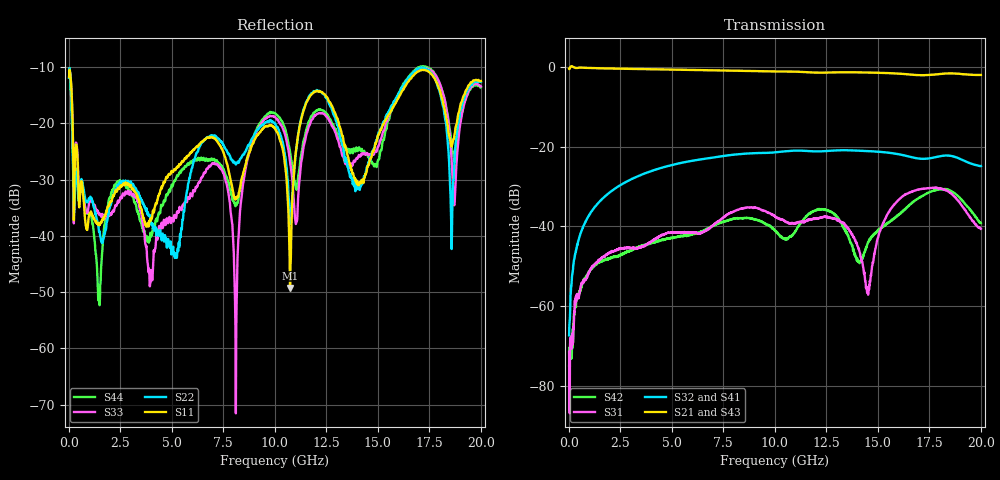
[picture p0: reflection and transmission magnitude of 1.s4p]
!Keysight Technologies,N5225A,MY51451420,A.10.40.12
!Date: Tuesday, October 13, 2015 09:32:39
!Correction: S11(Full 4 Port(1,2,3,4))
!S12(Full 4 Port(1,2,3,4))
!S13(Full 4 Port(1,2,3,4))
!S14(Full 4 Port(1,2,3,4))
!S21(Full 4 Port(1,2,3,4))
!S22(Full 4 Port(1,2,3,4))
!S23(Full 4 Port(1,2,3,4))
!S24(Full 4 Port(1,2,3,4))
!S31(Full 4 Port(1,2,3,4))
!S32(Full 4 Port(1,2,3,4))
!S33(Full 4 Port(1,2,3,4))
!S34(Full 4 Port(1,2,3,4))
!S41(Full 4 Port(1,2,3,4))
!S42(Full 4 Port(1,2,3,4))
!S43(Full 4 Port(1,2,3,4))
!S44(Full 4 Port(1,2,3,4))
!S4P File: Measurements: <S11,S12,S13,S14>,
!<S21,S22,S23,S24>,
!<S31,S32,S33,S34>,
!<S41,S42,S43,S44>:
# Hz S  dB  R 50
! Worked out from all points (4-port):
!   1999 points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, 20 MHz to 20 GHz, reference 50 ohm
!   strongest paths, dB at 20 MHz, 5.01 GHz, 10.01 GHz, 15.01 GHz, 20 GHz:
!     S21: -0.5, -0.7, -1.2, -1.5, -2.0
!     S43: -0.5, -0.7, -1.2, -1.5, -1.9
!     S32: -67.4, -24.6, -21.5, -21.3, -24.9
!     S41: -68.7, -24.6, -21.5, -21.3, -24.9
!     S31: -71.5, -41.6, -37.6, -42.8, -40.6
!     S42: -74.9, -43.0, -41.0, -41.1, -39.2
!   lowest |S11| = -49.3 dB at 10.74 GHz (marker M1), VSWR 1.01, Z = 50.1 - j0.322 ohm
!   |S11| at or under -10 dB: start of sweep to end of sweep
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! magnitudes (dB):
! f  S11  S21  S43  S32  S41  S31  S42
! 20 MHz  -11.8  -0.5  -0.5  -67.4  -68.7  -71.5  -74.9
! 1.47 GHz  -38.1  -0.4  -0.4  -34.0  -34.0  -48.6  -49.1
! 7.21 GHz  -23.2  -0.9  -0.9  -22.6  -22.6  -39.0  -39.4
! 8.11 GHz  -33.5  -1.0  -1.0  -22.0  -22.0  -36.0  -38.1
! 10.74 GHz  -49.3  -1.2  -1.2  -21.1  -21.1  -39.3  -42.7
! 11.84 GHz  -14.7  -1.4  -1.3  -21.2  -21.2  -38.3  -36.3
! 20 GHz  -12.4  -2.0  -1.9  -24.9  -24.9  -40.6  -39.2
